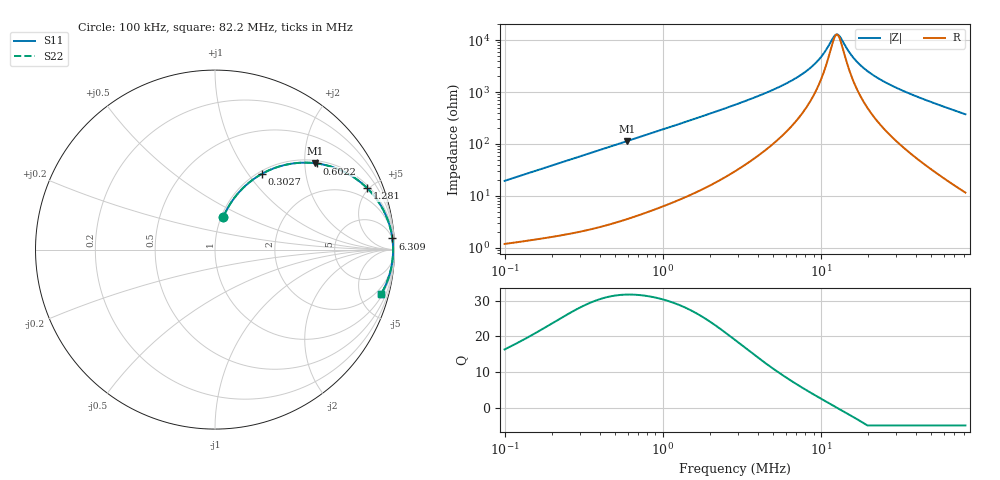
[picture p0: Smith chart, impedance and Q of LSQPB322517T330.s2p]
! LSQPB322517T330  S-PARAMETER MODEL  ( General Type )
! Model Generated by TAIYO YUDEN Corporation (http://www.ty-top.com)
! Version 2.0
! TAIYO YUDEN Control No. 100810NG22EB-FKC
! Copyright(c) 2009 TAIYO YUDEN CO.,LTD. All Rights Reserved.
! Product Description (link to TY-COMPAS)
! https://ds.yuden.co.jp/TYCOMPAS/or/detail?pn=LSQPB322517T330K&u=M
! Products Name : Inductors
! Characteristics :
!  Inductance : 33 uH , SRF(min) : 9.0 MHz , DC Resistance(max) : 1.008 Ohm
!  Rated Current : Saturation :470 mA , Temp Rise : 420 mA (40 degC)
!  Case Size : 3.2 x 2.5 / 0.126 x 0.098 [mm/inch] , Thickness : 1.7 / 0.068 [mm/inch]
!  (Conditions: Temperature = 25 degC , DC Bias Current/Voltage = 0A / 0V)
! External Node Assignments :
!  1  o---GGG---o  2
! GND o---------o GND
! Frequency Range : 0.1MHz  -  82.198079MHz  [ 402 STEP ]
# MHz S RI R 50
! Freq[MHz].  S11 Real  S11 Imag  S21 Real  S21 Imag  S12 Real  S12 Imag  S22 Real  S22 Imag
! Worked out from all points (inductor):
!   401 points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, 100 kHz to 82.2 MHz, reference 50 ohm
!   read as one part in series: L = 30.9 uH near 103.4 kHz
!   highest Q = 31.8 at 592.2 kHz (marker M1), where L = 30.4 uH
!   self-resonance near 12.55 MHz
!   S11 on the Smith chart (normalised r, x): 100 kHz: 1.02, +0.39; 302.7 kHz: 1.04, +1.16; 602.2 kHz: 1.07, +2.30; 1.281 MHz: 1.17, +4.89; 6.309 MHz: 5, +31; 82.2 MHz: 1.23, -7.48
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0.1  0.0471 0.1836  0.9529 -0.1836  0.9529 -0.1836  0.0471 0.1836
0.182952  0.1217 0.3057  0.8783 -0.3057  0.8783 -0.3057  0.1217 0.3057
0.302658  0.2602 0.4214  0.7398 -0.4214  0.7398 -0.4214  0.2602 0.4214
0.307779  0.2663 0.4248  0.7337 -0.4248  0.7337 -0.4248  0.2663 0.4248
0.592159  0.5595 0.4809  0.4405 -0.4809  0.4405 -0.4809  0.5595 0.4809
0.602179  0.5675 0.4799  0.4325 -0.4799  0.4325 -0.4799  0.5675 0.4799
0.947281  0.7582 0.4122  0.2418 -0.4122  0.2418 -0.4122  0.7582 0.4122
1.28129  0.8484 0.3417  0.1516 -0.3417  0.1516 -0.3417  0.8484 0.3417
2.867021  0.9616 0.1676  0.0384 -0.1676  0.0384 -0.1676  0.9616 0.1676
4.510077  0.9815 0.1002  0.0185 -0.1002  0.0185 -0.1002  0.9815 0.1002
6.308514  0.9881 0.0621  0.0119 -0.0621  0.0119 -0.0621  0.9881 0.0621
8.824095  0.9913 0.0305  0.00872 -0.0305  0.00872 -0.0305  0.9913 0.0305
10.26253  0.992 0.0174  0.00805 -0.0174  0.00805 -0.0174  0.992 0.0174
12.13741  0.9923 0.00341  0.00772 -0.00341  0.00772 -0.00341  0.9923 0.00341
12.76402  0.9923 -0.000763  0.0077 0.000763  0.0077 0.000763  0.9923 -0.000763
13.42298  0.9923 -0.00494  0.00772 0.00494  0.00772 0.00494  0.9923 -0.00494
15.6111  0.992 -0.0176  0.00799 0.0176  0.00799 0.0176  0.992 -0.0176
17.55672  0.9916 -0.0277  0.00845 0.0277  0.00845 0.0277  0.9916 -0.0277
21.11554  0.9903 -0.0443  0.00966 0.0443  0.00966 0.0443  0.9903 -0.0443
27.15873  0.9874 -0.0694  0.0126 0.0694  0.0126 0.0694  0.9874 -0.0694
44.18114  0.9747 -0.1306  0.0253 0.1306  0.0253 0.1306  0.9747 -0.1306
82.19808  0.9267 -0.2456  0.0733 0.2456  0.0733 0.2456  0.9267 -0.2456
